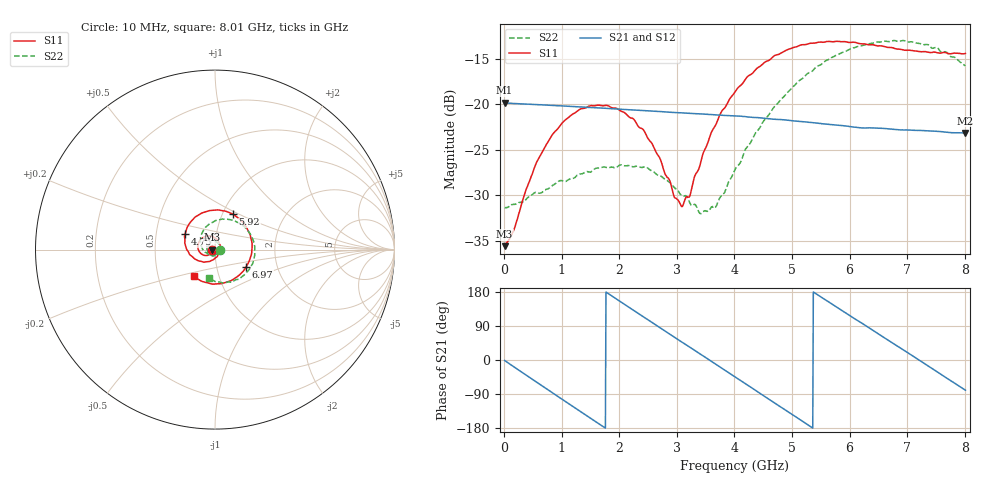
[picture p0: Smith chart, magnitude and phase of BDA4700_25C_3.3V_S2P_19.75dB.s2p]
!Agilent Technologies,E5071B,MY42404982,A.09.10
!Date: Mon Oct 20 18:11:21 2025
!Data & Calibration Information:
!Freq	S11:SOLT2(ON)	S21:SOLT2(ON)	S12:SOLT2(ON)	S22:SOLT2(ON)
# Hz S RI R 50
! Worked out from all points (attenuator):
!   801 points, 10 MHz to 8.01 GHz, reference 50 ohm
!   highest |S21| = -19.83 dB at 10 MHz (marker M1); lowest = -23.1 dB at 8.01 GHz (marker M2)
!   lowest |S11| = -35.6 dB at 10 MHz (marker M3), VSWR 1.03, Z = 48.4 - j0.105 ohm
!   |S11| at or under -10 dB: start of sweep to end of sweep
!   |S22| runs from -32.0 to -13.0 dB; largest |S21 - S12| = 0.0013
!   S11 on the Smith chart (normalised r, x): 10 MHz: 0.97, -0.00; 4.75 GHz: 0.70, +0.12; 5.92 GHz: 1.12, +0.46; 6.97 GHz: 1.39, -0.28; 8.01 GHz: 0.76, -0.23
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1e7  -0.0166 -0.00108  0.102 -0.0022  0.1019 -0.00234  0.0271 -0.000868
1.6e8  -0.0175 -0.00982  0.0968 -0.0293  0.0968 -0.0293  0.0271 -0.00772
4.1e8  -0.0262 -0.0243  0.0738 -0.0678  0.0738 -0.0678  0.021 -0.0223
7.1e8  -0.048 -0.0329  0.0286 -0.0949  0.0286 -0.095  0.00512 -0.0335
1.03e9  -0.0768 -0.0235  -0.0267 -0.0942  -0.0266 -0.0942  -0.0171 -0.0337
1.35e9  -0.0947 0.00441  -0.0722 -0.0644  -0.0722 -0.0644  -0.0376 -0.0176
2.08e9  -0.0526 0.0737  -0.0796 0.0496  -0.0796 0.0497  -0.029 0.0357
2.42e9  -0.00926 0.0718  -0.0375 0.0844  -0.0375 0.0844  -0.00265 0.0451
2.68e9  0.0178 0.0491  0.00323 0.0914  0.00307 0.0913  0.0156 0.0374
2.96e9  0.0285 0.0115  0.0449 0.0782  0.0448 0.0781  0.0279 0.021
3.1e9  0.0261 -0.00877  0.0623 0.0645  0.0619 0.0648  0.0301 0.00908
3.23e9  0.0188 -0.0255  0.0745 0.049  0.0746 0.0489  0.0286 -0.000142
3.54e9  -0.0169 -0.0594  0.0881 0.00368  0.0881 0.00353  0.0129 -0.0224
3.69e9  -0.0421 -0.0667  0.0853 -0.0189  0.0854 -0.0192  -0.000337 -0.0278
4.01e9  -0.1016 -0.0577  0.0616 -0.0606  0.0617 -0.0604  -0.034 -0.0272
4.75e9  -0.1671 0.0852  -0.0396 -0.0725  -0.0393 -0.0728  -0.0813 0.0601
5.35e9  -0.0658 0.2064  -0.0793 -0.00208  -0.0793 -0.00248  -0.0145 0.1513
5.92e9  0.1005 0.1969  -0.0437 0.0623  -0.044 0.062  0.1171 0.1558
6.68e9  0.2052 -0.00725  0.046 0.0571  0.0461 0.0571  0.2212 -0.00607
6.97e9  0.1738 -0.0952  0.0665 0.0283  0.0665 0.028  0.2063 -0.0835
7.48e9  0.0414 -0.1887  0.0632 -0.0327  0.0633 -0.0328  0.0989 -0.1794
8.01e9  -0.1186 -0.1487  0.0124 -0.0685  0.0127 -0.0685  -0.0359 -0.1584
